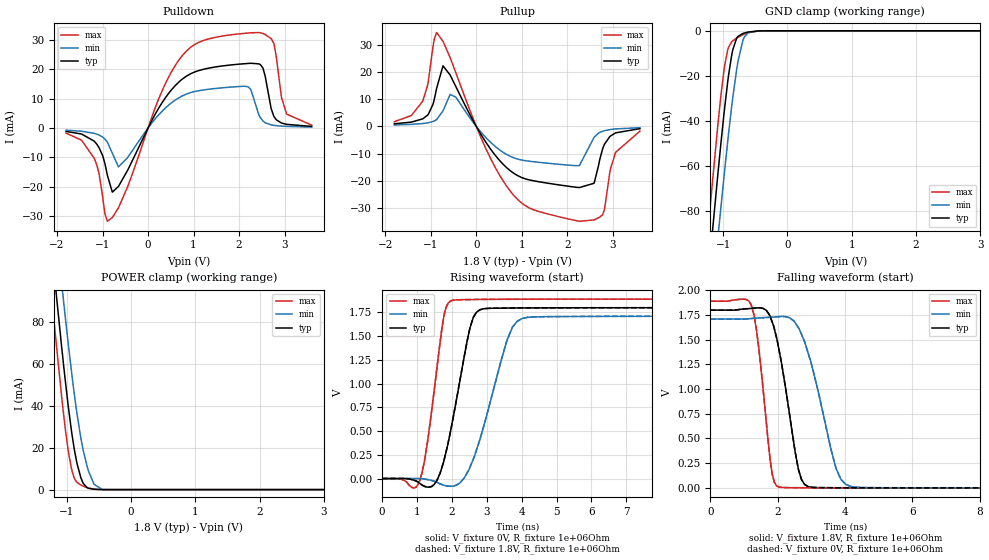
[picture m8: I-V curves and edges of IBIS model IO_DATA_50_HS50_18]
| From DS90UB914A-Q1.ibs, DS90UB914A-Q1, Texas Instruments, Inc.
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|   Model IO_DATA_50_HS50_18
[Model]  IO_DATA_50_HS50_18
Model_type   I/O
Polarity   Non-Inverting
Enable   Active-Low
Vinl =   0.63
Vinh =   1.17
Vmeas = 0.8V
|   typ   min   max
|   (nom)   (fast)   (slow)
C_comp   1.107pF   1.107pF   1.107pF
[Temperature Range]   25.000   105.00   -40.000
[Voltage Range]   1.800V   1.700V   1.900V
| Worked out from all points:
|   slope of the pulldown table from 0 to 0.27 V, typ, clamps not added: 35 ohm
|   slope of the pullup table from 0 to 0.27 V, typ, clamps not added: 37 ohm
|   GND clamp passes 1 mA (typ) near -0.67 V on its own axis
|   POWER clamp passes 1 mA (typ) near -0.68 V on its own axis
|   falling waveform, V_fixture 1.8V, R_fixture 1e+06Ohm: 20-80 % time 505ps typ, 718ps min, 343ps max; typ from 1.8 V to 0 V
|   rising waveform, V_fixture 0V, R_fixture 1e+06Ohm: 20-80 % time 549ps typ, 767ps min, 391ps max; typ from 0 V to 1.8 V
|   rising waveform, V_fixture 1.8V, R_fixture 1e+06Ohm: 20-80 % time 549ps typ, 768ps min, 391ps max; typ from 0 V to 1.8 V
|   falling waveform, V_fixture 0V, R_fixture 1e+06Ohm: 20-80 % time 505ps typ, 718ps min, 343ps max; typ from 1.8 V to 0 V
[Pulldown]
|   Voltage   I(typ)   I(min)   I(max)
-1.8V     -1.151mA   -721.1uA   -1.73mA
-1.184V   -4.457mA   -1.79mA    -10.3mA
-892.8mV  -16.14mA   -4.822mA   -31.85mA
-784.8mV  -21.89mA   -8.592mA   -30.57mA
-649.8mV  -19.94mA   -13.27mA   -27.23mA
711mV     16.19mA    10.63mA    23.93mA
2.266V    22.12mA    12.78mA    32.53mA
2.52V     20.59mA    2.471mA    32.32mA
2.817V    2.829mA    815uA      24.38mA
2.93V     1.726mA    663.8uA    10.47mA
3.044V    1.258mA    564.1uA    4.777mA
3.595V    561.6uA    334.1uA    989.3uA
[GND Clamp]
|   Voltage   I(typ)   I(min)   I(max)
-1.8V     -294.5mA   -316mA     -279mA
-1.228V   -108.2mA   -135.9mA   -86.66mA
-1.168V   -89.73mA   -117.9mA   -67.77mA
-1.082V   -63.6mA    -92.1mA    -41.63mA
-1.033V   -49.54mA   -77.98mA   -28.3mA
-979.2mV  -34.85mA   -62.72mA   -15.97mA
-930.6mV  -23mA      -49.56mA   -8.668mA
-871.2mV  -11.45mA   -34.54mA   -5.024mA
-768.6mV  -2.465mA   -13.49mA   -2.849mA
-693mV    -1.185mA   -4.278mA   -1.721mA
-450mV    -39.16uA   -30.07uA   -81.5uA
3.595V    0A         0A         0A
[Pullup]
|   Voltage   I(typ)   I(min)   I(max)
-1.8V     957.1uA    528.8uA    1.718mA
-1.179V   2.76mA     1.04mA     9.229mA
-871.2mV  14.03mA    2.503mA    34.58mA
-730.8mV  22.32mA    5.727mA    31.36mA
-450mV    14.72mA    10.77mA    19.82mA
225mV     -6.204mA   -4.374mA   -8.715mA
721.8mV   -16mA      -10.84mA   -23.32mA
2.266V    -22.55mA   -14.44mA   -34.99mA
2.585V    -20.98mA   -4.093mA   -34.49mA
2.774V    -8.356mA   -1.807mA   -32.57mA
3.06V     -2.385mA   -935.3uA   -9.572mA
3.595V    -841.5uA   -484.6uA   -1.75mA
[POWER Clamp]
|   Voltage   I(typ)   I(min)   I(max)
-1.8V     299.8mA    323.2mA    282.8mA
-1.217V   110.3mA    140.1mA    86.99mA
-1.19V    101.9mA    131.9mA    78.38mA
-1.076V   67.7mA     98.25mA    43.89mA
-1.044V   58.39mA    88.9mA     34.92mA
-973.8mV  39.52mA    69.31mA    18.28mA
-914.4mV  25.75mA    53.74mA    8.664mA
-779.4mV  5.662mA    24.62mA    2.183mA
-660.6mV  654.1uA    8.858mA    728.4uA
-574.2mV  160.2uA    2.529mA    194.7uA
-450mV    11.37uA    103.3uA    10.88uA
3.595V    0A         0A         0A
[Ramp]
R_load = 1e+06
|   typ   min   max
dV/dt_r   1.07991/5.4858e-10   1.02573/7.67494e-10   1.13396/3.9129e-10
dV/dt_f   1.07991/5.05064e-10   1.02572/7.1822e-10   1.13396/3.43297e-10
[Falling Waveform]
V_fixture = 1.8V
V_fixture_min = 1.71V
V_fixture_max = 1.89V
R_fixture = 1e+06Ohm
C_fixture = 0F
|   Time   V(typ)   V(min)   V(max)
0s        1.8V       1.71V      1.89V
1.212ns   1.817V     1.715V     1.855V
1.44ns    1.823V     1.721V     1.413V
1.836ns   1.68V      1.729V     141.4mV
2.035ns   1.405V     1.734V     8.609mV
2.705ns   85.93mV    1.556V     1.265mV
2.993ns   6.768mV    1.267V     904.4uV
3.733ns   1.334mV    197.3mV    599.2uV
4.009ns   1.144mV    38.04mV    520uV
10.05ns   91.3uV     212.7uV    49.35uV
[Rising Waveform]
V_fixture = 0V
V_fixture_min = 0V
V_fixture_max = 0V
R_fixture = 1e+06Ohm
C_fixture = 0F
|   Time   V(typ)   V(min)   V(max)
0s        36.48uV    131uV      10.52uV
1.08ns    -50.15mV   -941.6uV   -22.26mV
1.294ns   -89.4mV    -9.35mV    364.8mV
1.576ns   -17.94mV   -40.88mV   1.175V
1.775ns   190.9mV    -70.29mV   1.718V
1.965ns   501.8mV    -81.42mV   1.871V
2.615ns   1.698V     204.4mV    1.886V
3.575ns   1.796V     1.45V      1.888V
3.871ns   1.797V     1.656V     1.889V
10.05ns   1.8V       1.71V      1.89V
[Rising Waveform]
V_fixture = 1.8V
V_fixture_min = 1.71V
V_fixture_max = 1.89V
R_fixture = 1e+06Ohm
C_fixture = 0F
|   Time   V(typ)   V(min)   V(max)
0s        93.56uV    216.3uV    51uV
1.08ns    -49.97mV   -372.3uV   -21.61mV
1.294ns   -88.87mV   -10.89mV   365.6mV
1.576ns   -17.07mV   -40.66mV   1.175V
1.775ns   191.9mV    -69.79mV   1.719V
1.965ns   502.8mV    -80.66mV   1.871V
2.615ns   1.698V     205.8mV    1.886V
3.575ns   1.796V     1.452V     1.888V
3.871ns   1.797V     1.656V     1.889V
10.05ns   1.8V       1.71V      1.89V
[Falling Waveform]
|Gnd
V_fixture = 0V
V_fixture_min = 0V
V_fixture_max = 0V
R_fixture = 1e+06Ohm
C_fixture = 0F
|   Time   V(typ)   V(min)   V(max)
0s        1.8V       1.71V      1.89V
1.212ns   1.817V     1.715V     1.855V
1.44ns    1.823V     1.721V     1.412V
1.836ns   1.68V      1.729V     141.1mV
2.035ns   1.404V     1.734V     8.492mV
2.705ns   85.51mV    1.555V     1.202mV
2.993ns   6.615mV    1.266V     847.6uV
3.733ns   1.242mV    196.4mV    548.7uV
4.009ns   1.057mV    37.67mV    471uV
10.05ns   34.26uV    127.4uV    8.842uV
